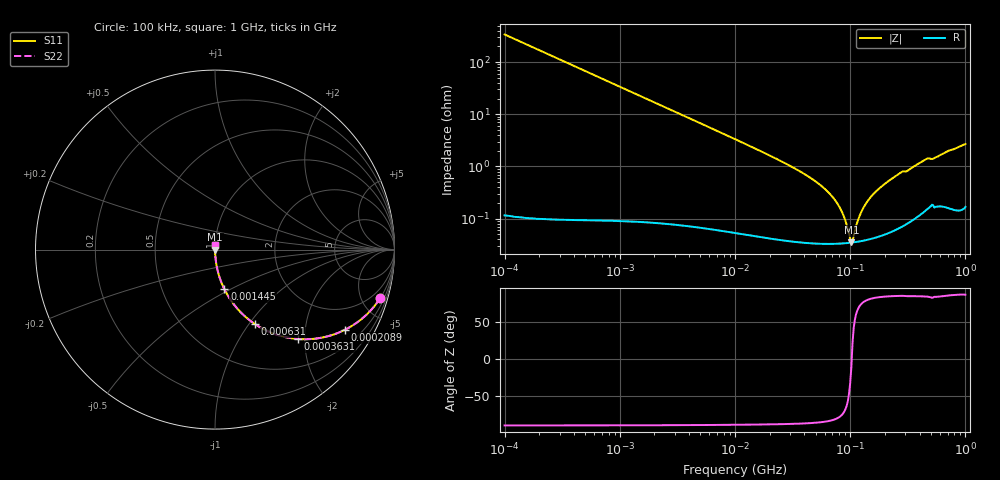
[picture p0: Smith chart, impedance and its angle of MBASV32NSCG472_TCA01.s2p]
! MBASV32NSCG472_TCA01  S-PARAMETER MODEL  ( Standard Model )
! Model Generated by TAIYO YUDEN Corporation (https://www.yuden.co.jp/en/)
! Version 1.0
! TAIYO YUDEN Control No. 250312
! Copyright(c) 2025 TAIYO YUDEN CO.,LTD. All Rights Reserved.
! Product Description (link to TY-COMPAS)
! https://ds.yuden.co.jp/TYCOMPAS/or/detail?pn=MBASV32NSCG472JTCA01&u=M
! Products Name : Multilayer Ceramic Capacitors
! Characteristics :
!  Capacitance : 4700 [pF] , Rated Voltage : 1000 [V] , TCC : CG / C0G
!  Case Size : 3.2 x 2.5 / 0.126 x 0.098 [mm/inch] , Thickness : 1.9 / 0.075 [mm/inch]
!  (Conditions: Temperature = 25 [degC] , DC Bias Voltage = 0 [V])
! External Node Assignments :
!  1  o---| |---o  2
! GND o---------o GND
! Frequency Range : 0.1MHz  -  1000MHz  [ 401 STEP ]
# MHZ S RI R 50
! Freq[MHz].  S11 Real  S11 Imag  S21 Real  S21 Imag  S12 Real  S12 Imag  S22 Real  S22 Imag
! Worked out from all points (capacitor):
!   401 points, 100 kHz to 1 GHz, reference 50 ohm
!   read as one part in series: C = 4.72 nF near 104.7 kHz
!   lowest |Z| = 35.6 mohm at 102.3 MHz (marker M1)
!   series resonance near 103.2 MHz, so ESL is about 500 pH
!   S11 on the Smith chart (normalised r, x): 100 kHz: 1.00, -6.75; 208.9 kHz: 1.00, -3.23; 363.1 kHz: 1.00, -1.86; 631 kHz: 1.00, -1.07; 1.445 MHz: 1.00, -0.47; 1 GHz: 1.00, +0.05
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0.1  0.9192 -0.2724  0.0808 0.2724  0.0808 0.2724  0.9192 -0.2724
0.20893  0.7228 -0.4473  0.2772 0.4473  0.2772 0.4473  0.7228 -0.4473
0.363078  0.4637 -0.4982  0.5363 0.4982  0.5363 0.4982  0.4637 -0.4982
0.467735  0.3427 -0.474  0.6573 0.474  0.6573 0.474  0.3427 -0.474
0.630957  0.223 -0.4154  0.777 0.4154  0.777 0.4154  0.223 -0.4154
1.44544  0.0525 -0.2211  0.9475 0.2211  0.9475 0.2211  0.0525 -0.2211
2.187762  0.024 -0.1504  0.976 0.1504  0.976 0.1504  0.024 -0.1504
10  0.00164 -0.0333  0.9984 0.0333  0.9984 0.0333  0.00164 -0.0333
46.77351  0.000369 -0.00574  0.9996 0.00574  0.9996 0.00574  0.000369 -0.00574
61.6595  0.000341 -0.00353  0.9997 0.00353  0.9997 0.00353  0.000341 -0.00353
75.85776  0.000335 -0.00206  0.9997 0.00206  0.9997 0.00206  0.000335 -0.00206
87.09636  0.000337 -0.00113  0.9997 0.00113  0.9997 0.00113  0.000337 -0.00113
97.72372  0.000344 -0.000371  0.9997 0.000371  0.9997 0.000371  0.000344 -0.000371
102.3293  0.000348 -7.23e-05  0.9997 7.23e-05  0.9997 7.23e-05  0.000348 -7.23e-05
107.1519  0.000353 0.000306  0.9996 -0.000306  0.9996 -0.000306  0.000353 0.000306
123.0269  0.000371 0.0012  0.9996 -0.0012  0.9996 -0.0012  0.000371 0.0012
138.0384  0.000393 0.00196  0.9996 -0.00196  0.9996 -0.00196  0.000393 0.00196
165.9587  0.000443 0.00323  0.9996 -0.00323  0.9996 -0.00323  0.000443 0.00323
218.7762  0.000566 0.00538  0.9994 -0.00538  0.9994 -0.00538  0.000566 0.00538
457.0882  0.00165 0.0138  0.9984 -0.0138  0.9984 -0.0138  0.00165 0.0138
537.0318  0.00183 0.0143  0.9982 -0.0143  0.9982 -0.0143  0.00183 0.0143
1000  0.00239 0.0268  0.9976 -0.0268  0.9976 -0.0268  0.00239 0.0268
